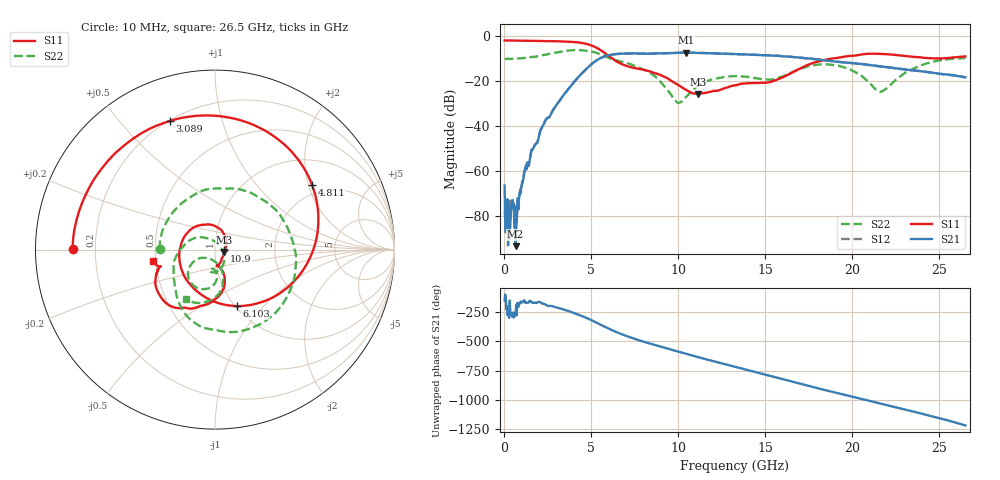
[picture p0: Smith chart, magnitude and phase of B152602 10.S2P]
!  2-Port S-parameters saved by WinCal
! VAR MeasName=S-Parameters (CALIBRATED_DATA) read from VNA (N5242A)
! VAR MeasDate=2016-1-5 16:26:54
! VAR NAME=B152602 10
! VAR FILENAME=B152602 10.S2P
! VAR DATE=2016-1-5 16:26:54
! VAR PHYS_PORTS=1,2
# Hz S DB R 50
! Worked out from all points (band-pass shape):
!   801 points, 10 MHz to 26.5 GHz, reference 50 ohm
!   highest |S21| = -7.44 dB at 10.44 GHz (marker M1); lowest = -93.2 dB at 639.1 MHz (marker M2)
!   |S21| within 3 dB of the highest: 5.375 GHz to 18.05 GHz (12.68 GHz wide, 108 % of centre)
!   lowest |S11| = -25.7 dB at 11.14 GHz (marker M3), VSWR 1.11, Z = 55.3 - j1.42 ohm
!   |S11| at or under -10 dB: 6.201 GHz to 18.86 GHz (12.66 GHz wide, 101 % of centre)
!   |S22| runs from -29.7 to -6.2 dB; largest |S21 - S12| = 0.0029
!   S11 on the Smith chart (normalised r, x): 10 MHz: 0.12, +0.00; 3.089 GHz: 0.20, +0.69; 4.811 GHz: 1.68, +2.11; 6.103 GHz: 1.02, -0.72; 10.9 GHz: 1.11, -0.01; 26.5 GHz: 0.48, -0.07
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1e7  -2.01 179.7  -66.36 -149.3  -77.67 177.9  -10.25 179.5
1.755625e8  -2.02 176.3  -72.35 87.3  -74.84 74.2  -10.18 170.1
6.391375e8  -2.07 166.8  -93.21 95.9  -84.05 96.8  -10.12 143.5
1.632512e9  -2.19 146.1  -50.39 -170.2  -50.25 -169.5  -9.35 87.4
3.089462e9  -2.39 109.4  -29.50 147.2  -29.50 147.1  -7.27 7.4
4.447075e9  -3.11 55.2  -16.64 78.4  -16.66 78.5  -6.35 -65.6
4.811312e9  -3.74 33.8  -13.88 55.5  -13.89 55.6  -6.76 -83.9
6.1027e9  -9.44 -69.1  -8.38 -37.3  -8.37 -37.3  -10.01 -133.8
7.129188e9  -13.58 -159.0  -7.79 -98.8  -7.78 -98.9  -12.24 -160.5
8.851038e9  -16.96 101.1  -7.72 -178.2  -7.73 -178.3  -19.29 140.1
9.910638e9  -21.40 45.0  -7.50 136.9  -7.50 137.0  -29.37 57.1
1.044044e10  -23.92 15.4  -7.44 114.5  -7.44 114.7  -27.03 -11.6
1.090401e10  -25.56 -5.2  -7.49 95.3  -7.49 95.3  -23.46 -39.4
1.11358e10  -25.67 -14.2  -7.55 85.9  -7.54 86.0  -22.13 -48.8
1.3255e10  -21.89 -70.5  -8.04 2.8  -8.03 2.8  -17.86 -95.3
1.547354e10  -20.00 -75.5  -8.76 -82.6  -8.72 -82.6  -19.15 -93.0
1.769208e10  -12.12 -82.7  -10.16 -168.3  -10.12 -168.2  -13.08 -101.1
1.984439e10  -8.87 -114.5  -11.99 113.4  -11.96 113.0  -14.80 -143.9
2.150001e10  -7.93 -139.0  -13.43 52.6  -13.40 52.2  -24.61 -123.8
2.209604e10  -8.16 -146.8  -13.99 31.0  -13.95 30.5  -22.40 -82.6
2.414901e10  -9.72 -162.1  -15.83 -44.3  -15.85 -44.6  -12.52 -83.3
2.65e10  -9.07 -169.8  -18.34 -138.8  -18.37 -138.9  -9.90 -120.3
